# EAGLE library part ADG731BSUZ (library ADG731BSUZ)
ADG731BSUZ, Multiplexer Single 32:1, 3, 5V, 48-Pin, TQFP Source: Datasheet
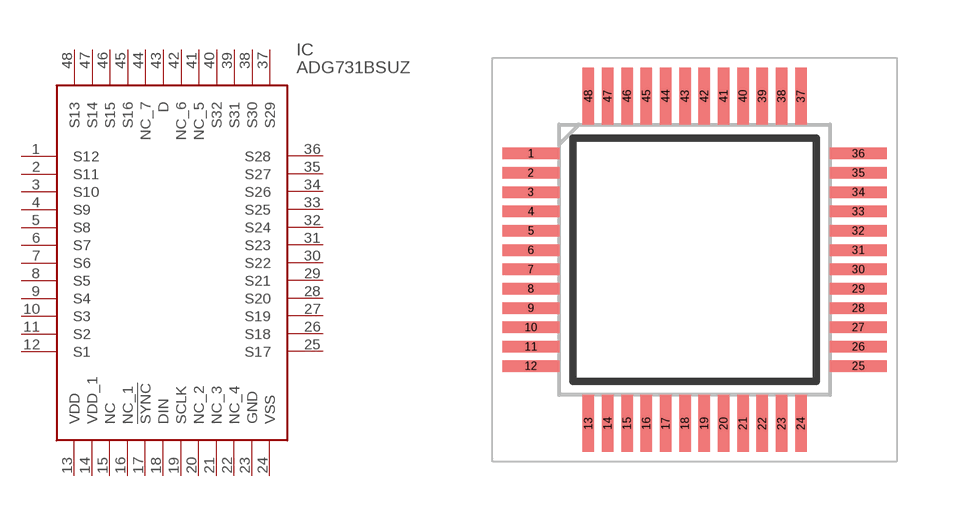
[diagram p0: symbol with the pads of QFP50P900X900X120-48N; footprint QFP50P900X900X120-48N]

Designator prefix IC

## ADG731BSUZ (Description: ADG731BSUZ, Multiplexer Single 32:1, 3, 5V, 48-Pin, TQFP; Height: 1.2mm; Manufacturer_Name: Analog Devices; Manufacturer_Part_Number: ADG731BSUZ; Mouser_Part_Number: 584-ADG731BSUZ; Mouser_Price-Stock: https://www.mouser.com/Search/Refine.aspx?Keyword=584-ADG731BSUZ)  [QFP50P900X900X120-48N]
1  S12
2  S11
3  S10
4  S9
5  S8
6  S7
7  S6
8  S5
9  S4
10  S3
11  S2
12  S1
13  VDD  pwr
14  VDD_1  pwr
15  NC  nc
16  NC_1
17  !SYNC
18  DIN  in
19  SCLK  in
20  NC_2
21  NC_3
22  NC_4
23  GND  pwr
24  VSS  pwr
25  S17
26  S18
27  S19
28  S20
29  S21
30  S22
31  S23
32  S24
33  S25
34  S26
35  S27
36  S28
37  S29
38  S30
39  S31
40  S32
41  NC_5
42  NC_6
43  D
44  NC_7
45  S16
46  S15
47  S14
48  S13

## Footprint QFP50P900X900X120-48N (pad centres in mm)
SU-48 (TQFP)
smd 1.475 x 0.3: 1 -4.238,2.75; 2 -4.238,2.25; 3 -4.238,1.75; 4 -4.238,1.25; 5 -4.238,0.75; 6 -4.238,0.25; 7 -4.238,-0.25; 8 -4.238,-0.75; 9 -4.238,-1.25; 10 -4.238,-1.75; 11 -4.238,-2.25; 12 -4.238,-2.75; 25 4.238,-2.75; 26 4.238,-2.25; 27 4.238,-1.75; 28 4.238,-1.25; 29 4.238,-0.75; 30 4.238,-0.25; 31 4.238,0.25; 32 4.238,0.75; 33 4.238,1.25; 34 4.238,1.75; 35 4.238,2.25; 36 4.238,2.75
smd 0.3 x 1.475: 13 -2.75,-4.238; 14 -2.25,-4.238; 15 -1.75,-4.238; 16 -1.25,-4.238; 17 -0.75,-4.238; 18 -0.25,-4.238; 19 0.25,-4.238; 20 0.75,-4.238; 21 1.25,-4.238; 22 1.75,-4.238; 23 2.25,-4.238; 24 2.75,-4.238; 37 2.75,4.238; 38 2.25,4.238; 39 1.75,4.238; 40 1.25,4.238; 41 0.75,4.238; 42 0.25,4.238; 43 -0.25,4.238; 44 -0.75,4.238; 45 -1.25,4.238; 46 -1.75,4.238; 47 -2.25,4.238; 48 -2.75,4.238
